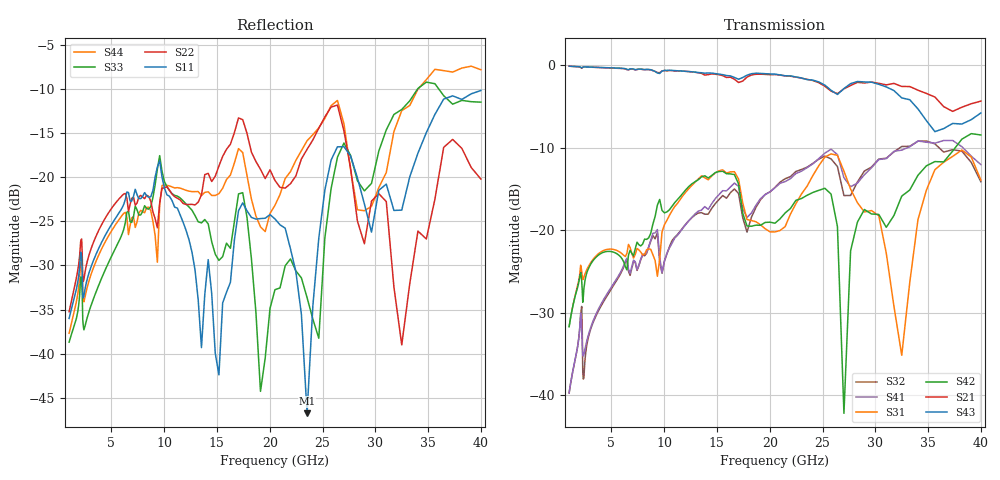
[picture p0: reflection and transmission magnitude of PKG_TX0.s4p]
! Created Mon Sep 18 16:13:13 2017
# hz S ma R 50
! 4 Port Network Data from SP1.SP block
! freq  magS11  angS11  magS12  angS12  magS13  angS13  magS14  angS14
!  magS21  angS21  magS22  angS22  magS23  angS23  magS24  angS24
!  magS31  angS31  magS32  angS32  magS33  angS33  magS34  angS34
!  magS41  angS41  magS42  angS42  magS43  angS43  magS44  angS44
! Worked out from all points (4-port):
!   161 points, 1 GHz to 40 GHz, reference 50 ohm
!   strongest paths, dB at 1 GHz, 2.515 GHz, 6.325 GHz, 15.91 GHz, 40 GHz:
!     S43: -0.1, -0.2, -0.4, -1.2, -5.8
!     S21: -0.1, -0.2, -0.4, -1.5, -4.3
!     S42: -31.7, -26.0, -24.4, -13.1, -8.4
!     S31: -31.7, -25.2, -23.2, -13.1, -13.9
!     S41: -39.7, -34.3, -23.7, -15.2, -12.0
!     S32: -39.7, -35.6, -23.9, -16.1, -14.1
!   lowest |S11| = -46.8 dB at 23.54 GHz (marker M1), VSWR 1.01, Z = 50.4 - j0.238 ohm
!   |S11| at or under -10 dB: start of sweep to end of sweep
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1e9  0.01583 54.6  0.9886 -17.8  0.02612 67.9  0.01035 -111.8
     0.9886 -17.8  0.01728 35.9  0.01032 -111.5  0.02606 74.0
     0.02612 67.9  0.01032 -111.5  0.01162 46.9  0.9892 -16.8
     0.01035 -111.8  0.02606 74.0  0.9892 -16.8  0.01304 29.1
1.074796e10  0.07366 -66.7  0.9298 174.3  0.1316 145.5  0.08341 88.9
             0.9298 174.3  0.08007 -112.0  0.08667 99.0  0.14 34.5
             0.1316 145.5  0.08667 99.0  0.08071 -58.9  0.9326 -175.5
             0.08341 88.9  0.14 34.5  0.9326 -175.5  0.08804 -105.5
1.784881e10  0.0644 143.6  0.849 56.5  0.1163 -36.6  0.1197 -57.3
             0.849 56.5  0.1769 -156.9  0.09753 -34.8  0.1063 -42.4
             0.1163 -36.6  0.09753 -34.8  0.05909 -160.1  0.8717 71.7
             0.1197 -57.3  0.1063 -42.4  0.8717 71.7  0.1025 -164.2
2.353769e10  0.004591 -30.9  0.8251 -49.2  0.1853 126.0  0.2399 -147.2
             0.8251 -49.2  0.1437 -132.2  0.2415 -128.1  0.1631 -45.5
             0.1853 126.0  0.2415 -128.1  0.02077 -75.4  0.8199 -29.0
             0.2399 -147.2  0.1631 -45.5  0.8199 -29.0  0.1608 -122.3
2.702969e10  0.1487 -41.3  0.7202 -100.4  0.2286 23.6  0.2087 119.5
             0.7202 -100.4  0.1827 132.5  0.1626 146.7  0.007781 25.0
             0.2286 23.6  0.1626 146.7  0.156 -38.2  0.7239 -77.5
             0.2087 119.5  0.007781 25.0  0.7239 -77.5  0.2009 146.5
3.250455e10  0.06503 -155.5  0.7454 154.7  0.0175 165.4  0.3065 40.8
             0.7454 154.7  0.01121 151.8  0.3224 70.8  0.1613 155.0
             0.0175 165.4  0.3224 70.8  0.2416 -101.8  0.6353 174.6
             0.3065 40.8  0.1613 155.0  0.6353 174.6  0.2381 -173.8
4e10  0.3097 -34.9  0.6075 26.2  0.2017 -18.5  0.2504 -137.3
      0.6075 26.2  0.09751 -27.1  0.1972 -94.6  0.3787 24.9
      0.2017 -18.5  0.1972 -94.6  0.266 18.9  0.515 79.2
      0.2504 -137.3  0.3787 24.9  0.515 79.2  0.4058 24.9
